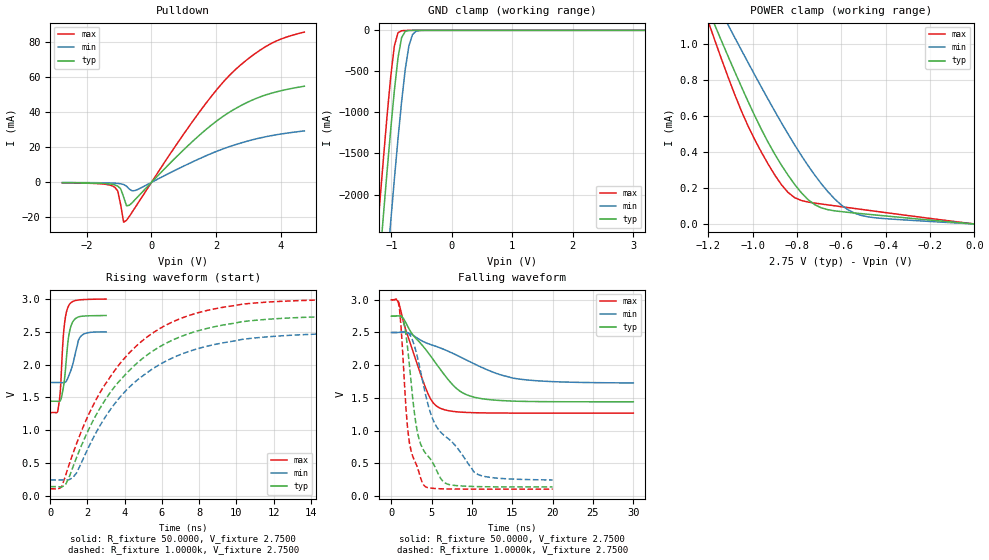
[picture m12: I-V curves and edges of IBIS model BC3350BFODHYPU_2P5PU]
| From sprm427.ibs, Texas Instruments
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|   Model BC3350BFODHYPU_2P5PU
[Model]   BC3350BFODHYPU_2P5PU
Model_type   I/O_open_drain
Polarity   Non-Inverting
Enable   Active-Low
Vinl =   0.7500V
Vinh =   1.7500V
Vmeas =   1.2500V
Cref =  15.0000pF
Rref = 100.0000M
Vref =  0.000V
C_comp   2.5179pF   2.5239pF   3.1043pF
[Temperature Range]   25.0000   0.1250k   -40.0000
[Voltage Range]   2.7500V   2.5000V   3.0000V
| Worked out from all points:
|   slope of the pulldown table from 0 to 0.412 V, typ, clamps not added: 52.2 ohm
|   GND clamp passes 1 mA (typ) near -0.67 V on its own axis
|   POWER clamp passes 1 mA (typ) near -1.14 V on its own axis
|   rising waveform, R_fixture 50.0000, V_fixture 2.7500: 20-80 % time 293ps typ, 424ps min, 235ps max; typ from 1.44 V to 2.75 V
|   rising waveform, R_fixture 1.0000k, V_fixture 2.7500: 20-80 % time 4.09ns typ, 4.17ns min, 3.93ns max; typ from 0.139 V to 2.75 V
|   falling waveform, R_fixture 50.0000, V_fixture 2.7500: 20-80 % time 5.07ns typ, 8.6ns min, 2.86ns max; typ from 2.75 V to 1.44 V
|   falling waveform, R_fixture 1.0000k, V_fixture 2.7500: 20-80 % time 2.15ns typ, 5.04ns min, 1.18ns max; typ from 2.75 V to 0.139 V
[Pulldown]
| voltage   I(typ)   I(min)   I(max)
-2.75V    -196uA     -89uA      -273uA
-1.13V    -1.446mA   -462.6uA   -2.767mA
-1.04V    -2.119mA   -590.9uA   -4.942mA
-950mV    -3.685mA   -805.6uA   -12.8mA
-860mV    -8.253mA   -1.217mA   -22.69mA
-770mV    -13.34mA   -2.137mA   -21.65mA
-680mV    -13.04mA   -3.916mA   -19.29mA
-410mV    -7.97mA    -3.938mA   -11.68mA
1.21V     22.34mA    11.17mA    33.18mA
2.38V     39.69mA    20.21mA    60.46mA
3.55V     49.97mA    26.1mA     77.65mA
4.72V     54.82mA    29.33mA    85.66mA
[GND_clamp]
| voltage   I(typ)   I(min)   I(max)
-2.75V    -17.91A    -19.01A    -17.27A
-1.25V    -3.342A    -4.502A    -2.647A
-1.19V    -2.789A    -3.947A    -2.094A
-1.13V    -2.244A    -3.398A    -1.555A
-1.01V    -1.205A    -2.328A    -562.6mA
-950mV    -733.6mA   -1.814A    -190.1mA
-890mV    -336.3mA   -1.323A    -29.07mA
-830mV    -88.4mA    -867.9mA   -5.356mA
-770mV    -13.2mA    -475.4mA   -1.526mA
-710mV    -1.913mA   -190.9mA   -466.5uA
-590mV    -127.7uA   -10.7mA    -150.5uA
3.2V      0A         0A         0A
[POWER_clamp]
| voltage   I(typ)   I(min)   I(max)
-2.73V    5.918mA    5.09mA     6.921mA
-1.2V     1.189mA    1.315mA    1.123mA
-1.17V    1.101mA    1.244mA    1.017mA
-1.11V    928.2uA    1.102mA    812.8uA
-1.08V    843.2uA    1.032mA    716uA
-990mV    599.2uA    825.4uA    467uA
-870mV    326.4uA    561.1uA    217.7uA
-810mV    218.9uA    437.6uA    145.6uA
-720mV    107uA      271.5uA    115.8uA
-600mV    68.28uA    105.2uA    95.65uA
-510mV    57.19uA    47.27uA    80.82uA
0V        270.1pA    1.544nA    291.2pA
[Ramp]
| variable   typ   min   max
dV/dt_r   1.2903m/1.5082n  0.5181m/2.0212n   2.4515m/0.3281n
dV/dt_f   0.7856/5.0194n   0.4625/8.5182n   1.0392/2.8274n
R_load = 50.0000
[Rising Waveform]
R_fixture = 50.0000
V_fixture = 2.7500
V_fixture_min = 2.5000
V_fixture_max = 3.0000
| time   V(typ)   V(min)   V(max)
0s        1.44V      1.726V     1.268V
424.2ps   1.438V     1.726V     1.322V
545.5ps   1.45V      1.725V     1.621V
666.7ps   1.595V     1.723V     2.289V
727.3ps   1.694V     1.724V     2.52V
818.2ps   1.931V     1.733V     2.728V
969.7ps   2.39V      1.813V     2.886V
1.212ns   2.653V     2.009V     2.961V
1.636ns   2.734V     2.429V     2.987V
3ns       2.747V     2.498V     2.998V
[Rising Waveform]
R_fixture = 1.0000k
V_fixture = 2.7500
V_fixture_min = 2.5000
V_fixture_max = 3.0000
| time   V(typ)   V(min)   V(max)
0s        139.1mV    241.5mV    106mV
606.1ps   133mV      241.5mV    132.4mV
808.1ps   162.6mV    239.3mV    295.9mV
1.212ns   434.2mV    277.6mV    639.7mV
2.222ns   1.102V     833.8mV    1.334V
3.434ns   1.654V     1.393V     1.899V
4.646ns   2.017V     1.757V     2.289V
6.263ns   2.33V      2.059V     2.607V
10.51ns   2.659V     2.39V      2.925V
20ns      2.747V     2.493V     2.998V
[Falling Waveform]
R_fixture = 50.0000
V_fixture = 2.7500
V_fixture_min = 2.5000
V_fixture_max = 3.0000
| time   V(typ)   V(min)   V(max)
0s        2.75V      2.5V       3V
909.1ps   2.753V     2.502V     2.963V
1.818ns   2.645V     2.5V       2.527V
4.242ns   2.243V     2.345V     1.655V
5.152ns   2.093V     2.304V     1.431V
6.061ns   1.938V     2.264V     1.343V
8.485ns   1.605V     2.13V      1.284V
11.21ns   1.489V     1.967V     1.272V
16.67ns   1.447V     1.777V     1.268V
30ns      1.441V     1.729V     1.268V
[Falling Waveform]
R_fixture = 1.0000k
V_fixture = 2.7500
V_fixture_min = 2.5000
V_fixture_max = 3.0000
| time   V(typ)   V(min)   V(max)
0s        2.75V      2.5V       3V
1.01ns    2.762V     2.503V     2.86V
1.616ns   2.618V     2.51V      1.742V
2.222ns   2.027V     2.476V     831.2mV
3.03ns    1.118V     2.223V     503mV
4.04ns    691.1mV    1.664V     164.8mV
5.657ns   380.7mV    1.05V      114.6mV
6.869ns   188mV      895.4mV    109.8mV
10.3ns    146mV      362.1mV    106.5mV
20ns      139.3mV    246.8mV    106mV
